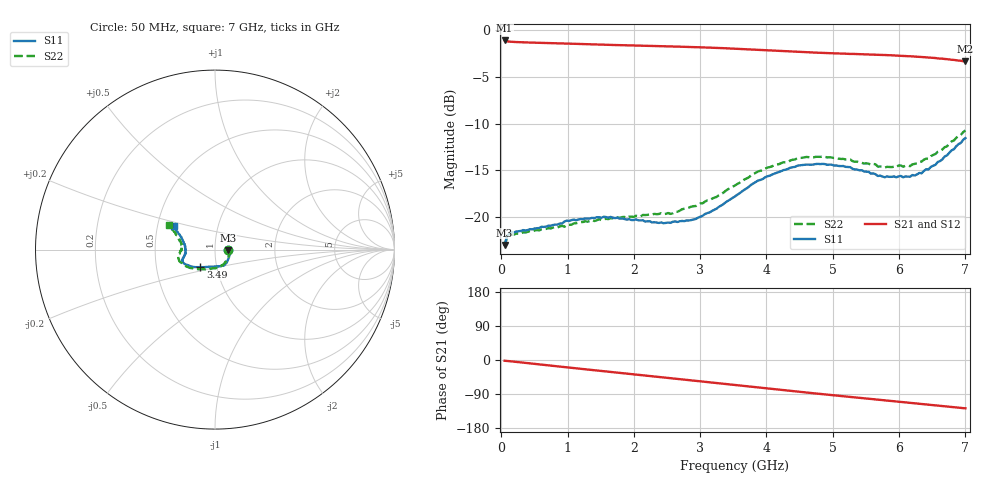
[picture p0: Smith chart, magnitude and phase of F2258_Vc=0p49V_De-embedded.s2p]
! Integrated Device Technology
! Corporate Headquarters
! 6024 Silver Creek Valley Road
! San Jose, CA 95138  USA
! Phone:  1-408-284-8200
! Toll Free:  1-800-223-1366
! Webpage:  http://www.idt.com/
! Timing and RF Division
! 515 Groton Road, Suite 102
! Westford, MA 01886-6024
! Device:  F2258
! Description: Voltage Variable RF Attenuator
! Frequency:  50.0 -  6000.00 MHz
! Package:  3x3 mm Thin QFN Plastic Package: 16 pin
! Ports:  2 RF, 2 DC
!  Pin  1  = NC
!  Pin  2  = NC
!  Pin  3  = RF2  = Port 2
!  Pin  4  = GND
!  Pin  5  = Vdd
!  Pin  6  = NC
!  Pin  7  = VCTRL
!  Pin  8  = NC
!  Pin  9  = GND
!  Pin 10  = RF1  = Port 1
!  Pin 11  = NC
!  Pin 12  = NC
!  Pin 13  = NC
!  Pin 14  = NC
!  Pin 15  = NC
!  Pin 16  = NC
! Vcntrl:  0.490 Volts
! Vdd:  +3.300 Volts
! Current:  1.101 mA
! Data:  The device was measured on a the F2258 evaluation board which has
!  individual transmission lines to the RF pins.  Data was collected
!  using a calibrated network analyzer.  The evaluation board was
!  de-embedded using a TRL calibration technique.
!  The reference plane is the edge of the package pin.
! Misc:  SN 10
!  Action Tracker AT0285
! Date Measured:  2014-12-10
! Date:  2016-01-13  MJV
! Note:
!  Integrated Device Technology supplies this data as a sample of measured
!  data at the package pin for this product.  Your particular data for this
!  product may vary.
!  Data was taken at 25 degrees C.
!  Integrated Device Technology reserves the right to change this data at anytime.
!Freq_(GHz)  S11M_(dB)  S11P_(deg)  S21M_(dB)  S21P_(deg)  S12M_(dB)  S12P_(deg)  S22M_(dB)  S22P_(deg)
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# GHz S dB R 50
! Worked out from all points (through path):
!   201 points, 50 MHz to 7 GHz, reference 50 ohm
!   highest |S21| = -1.09 dB at 50 MHz (marker M1); lowest = -3.3 dB at 7 GHz (marker M2)
!   group delay of S21, straight-line fit = 50.5 ps
!   lowest |S11| = -23.0 dB at 50 MHz (marker M3), VSWR 1.15, Z = 57.6 - j0.442 ohm
!   |S11| at or under -10 dB: start of sweep to end of sweep
!   |S22| runs from -23.1 to -10.7 dB; largest |S21 - S12| = 0.00058
!   S11 on the Smith chart (normalised r, x): 50 MHz: 1.15, -0.01; 3.49 GHz: 0.84, -0.17; 7 GHz: 0.61, +0.17
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0.05  -22.98 -3.1  -1.09 -2.0  -1.09 -2.0  -23.11 -3.1
0.08475  -22.07 -5.0  -1.18 -2.5  -1.18 -2.5  -22.22 -5.0
0.15425  -21.62 -7.9  -1.23 -3.7  -1.23 -3.7  -21.87 -8.6
0.71025  -20.91 -32.3  -1.37 -14.1  -1.37 -14.1  -21.18 -35.6
1.2315  -20.23 -52.7  -1.48 -23.8  -1.48 -23.8  -20.52 -59.5
1.6485  -19.97 -63.8  -1.57 -31.5  -1.57 -31.4  -20.12 -72.5
2.37825  -20.62 -83.3  -1.70 -44.8  -1.70 -44.8  -19.66 -91.0
2.552  -20.61 -89.1  -1.73 -48.0  -1.73 -48.0  -19.65 -96.3
2.93425  -20.19 -105.6  -1.81 -55.1  -1.81 -55.1  -18.81 -109.9
3.247  -19.09 -119.2  -1.89 -61.0  -1.89 -61.0  -17.83 -122.3
3.49025  -17.93 -129.7  -1.96 -65.6  -1.96 -65.6  -16.74 -131.6
3.525  -17.78 -130.7  -1.97 -66.2  -1.97 -66.2  -16.61 -133.1
4.0115  -15.63 -146.0  -2.15 -75.3  -2.15 -75.3  -14.70 -149.0
4.46325  -14.51 -155.1  -2.31 -83.4  -2.31 -83.4  -13.71 -160.3
4.7065  -14.37 -158.4  -2.38 -87.7  -2.39 -87.7  -13.60 -164.7
5.2625  -14.65 -165.2  -2.53 -97.4  -2.54 -97.4  -13.82 -173.0
5.6795  -15.60 -171.4  -2.62 -104.6  -2.62 -104.6  -14.59 -178.6
5.85325  -15.69 -175.6  -2.67 -107.8  -2.68 -107.8  -14.63 176.7
6.166  -15.67 176.3  -2.78 -113.3  -2.78 -113.3  -14.55 170.6
6.33975  -15.31 169.6  -2.86 -116.4  -2.87 -116.4  -14.04 166.1
6.722  -13.39 156.8  -3.09 -123.1  -3.10 -123.1  -12.43 156.9
7  -11.53 150.7  -3.34 -127.4  -3.34 -127.4  -10.71 151.9
